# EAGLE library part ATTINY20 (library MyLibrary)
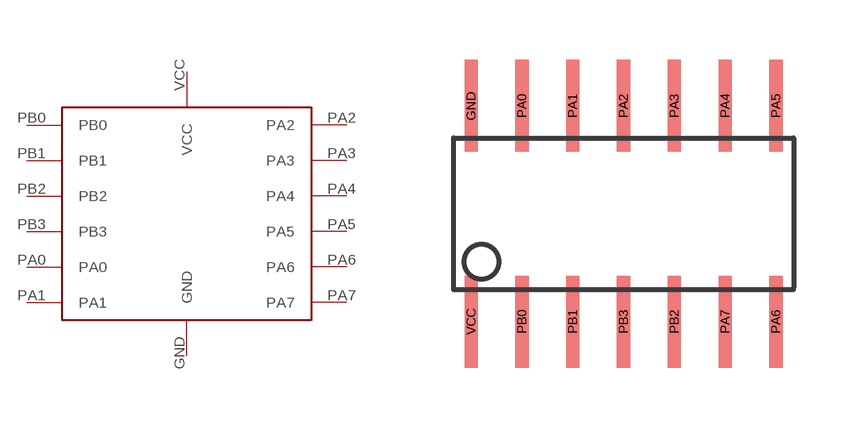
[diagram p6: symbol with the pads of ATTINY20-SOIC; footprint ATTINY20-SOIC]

Designator prefix -

## ATTINY20  [ATTINY20-SOIC]
GND  GND
PA0  PA0
PA1  PA1
PA2  PA2
PA3  PA3
PA4  PA4
PA5  PA5
PA6  PA6
PA7  PA7
PB0  PB0
PB1  PB1
PB2  PB2
PB3  PB3
VCC  VCC

## Footprint ATTINY20-SOIC (pad centres in mm)
smd 0.33 x 2.3: GND -3.81,2.7; PA0 -2.54,2.7; PA1 -1.27,2.7; PA2 0,2.7; PA3 1.27,2.7; PA4 2.54,2.7; PA5 3.81,2.7; PA6 3.81,-2.7; PA7 2.54,-2.7; PB0 -2.54,-2.7; PB1 -1.27,-2.7; PB2 1.27,-2.7; PB3 0,-2.7; VCC -3.81,-2.7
